DATA_BLOCK "Demo1"
TITLE =
VERSION : 0.1


  STRUCT
   str1 : STRING  [254 ] := '123 ABCDEFGH$R';	//write $$ to insert one single $; write $R to insert <CR> (0d hex)
  END_STRUCT ;
BEGIN
   str1 := '123 ABCDEFGH$R';
END_DATA_BLOCK

